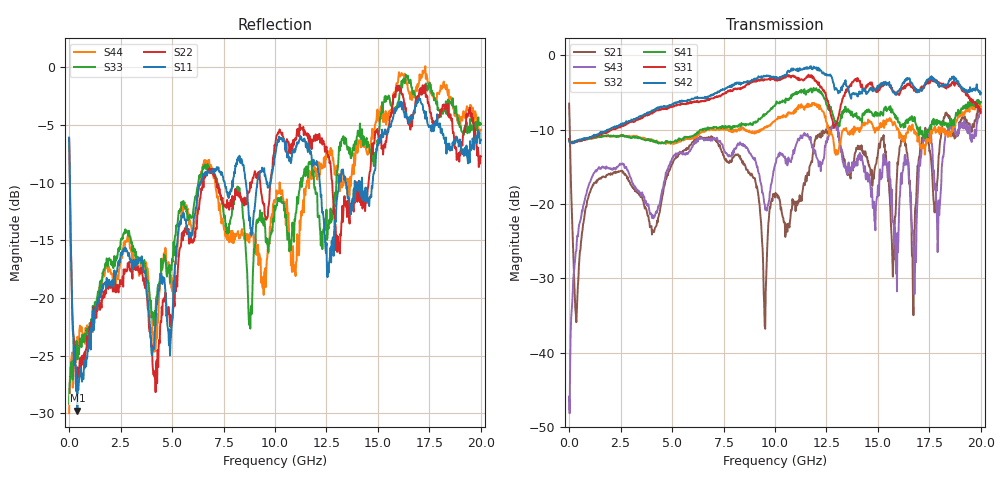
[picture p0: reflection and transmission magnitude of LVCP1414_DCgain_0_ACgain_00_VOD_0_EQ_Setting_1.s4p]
!Agilent Technologies,N5230A,MY46400459,A.07.50.48
!Agilent N5230A: A.07.50.48
!Date: Tuesday, April 17, 2012 18:33:44
!Correction: S11(Full 4 Port(1,2,3,4))
!S12(Full 4 Port(1,2,3,4))
!S13(Full 4 Port(1,2,3,4))
!S14(Full 4 Port(1,2,3,4))
!S21(Full 4 Port(1,2,3,4))
!S22(Full 4 Port(1,2,3,4))
!S23(Full 4 Port(1,2,3,4))
!S24(Full 4 Port(1,2,3,4))
!S31(Full 4 Port(1,2,3,4))
!S32(Full 4 Port(1,2,3,4))
!S33(Full 4 Port(1,2,3,4))
!S34(Full 4 Port(1,2,3,4))
!S41(Full 4 Port(1,2,3,4))
!S42(Full 4 Port(1,2,3,4))
!S43(Full 4 Port(1,2,3,4))
!S44(Full 4 Port(1,2,3,4))
!S4P File: Measurements: <S11,S12,S13,S14>,
!<S21,S22,S23,S24>,
!<S31,S32,S33,S34>,
!<S41,S42,S43,S44>:
# Hz S  dB  R 50
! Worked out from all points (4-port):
!   801 points, 300 kHz to 20 GHz, reference 50 ohm
!   strongest paths, dB at 300 kHz, 5 GHz, 10 GHz, 15 GHz, 20 GHz:
!     S42: -11.4, -6.6, -3.0, -4.2, -5.1
!     S31: -11.2, -6.9, -3.4, -4.9, -7.7
!     S41: -11.3, -11.6, -6.8, -7.8, -6.3
!     S32: -11.4, -11.8, -8.9, -9.9, -6.9
!     S43: -45.9, -13.9, -14.8, -17.5, -7.3
!     S21: -6.5, -14.7, -19.1, -13.2, -7.2
!   lowest |S11| = -29.8 dB at 400.3 MHz (marker M1), VSWR 1.07, Z = 53 + j1.51 ohm
!   |S11| at or under -10 dB: 37.79 MHz to 6.375 GHz (6.337 GHz wide, 198 % of centre); 8.588 GHz to 9.141 GHz (553.8 MHz wide, 6.25 % of centre); 12.17 GHz to 13.11 GHz (934.2 MHz wide, 7.39 % of centre)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
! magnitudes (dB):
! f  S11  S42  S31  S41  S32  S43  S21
! 300 kHz  -6.1  -11.4  -11.2  -11.3  -11.4  -45.9  -6.5
! 400.3 MHz  -29.8  -11.5  -11.5  -11.5  -11.5  -24.2  -32.7
! 9.975 GHz  -7.7  -3.0  -3.3  -6.8  -8.9  -14.9  -18.6
! 12.75 GHz  -15.1  -2.9  -8.4  -7.4  -10.6  -9.7  -9.9
! 14.03 GHz  -10.0  -5.5  -3.1  -8.5  -9.8  -13.9  -12.1
! 16.8 GHz  -3.5  -4.4  -4.5  -8.8  -10.2  -28.8  -21.0
! 20 GHz  -6.3  -5.1  -7.7  -6.3  -6.9  -7.3  -7.2
